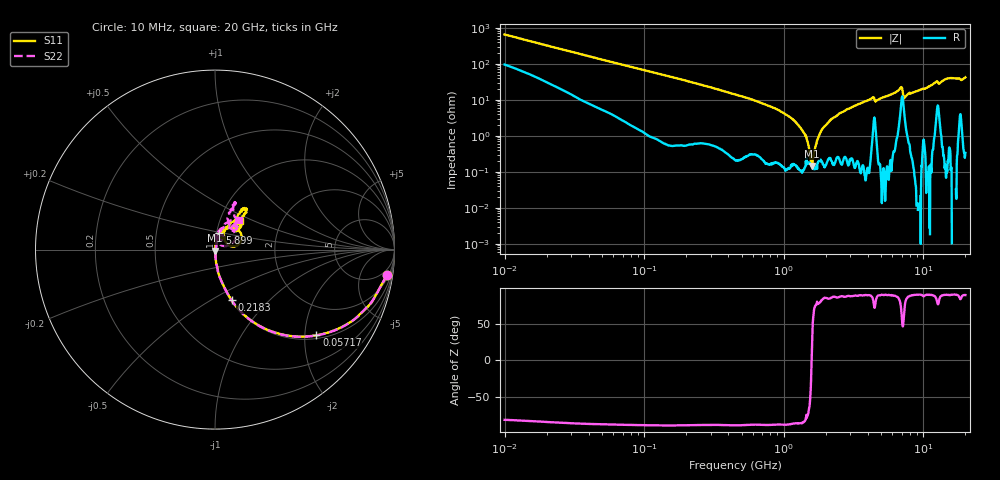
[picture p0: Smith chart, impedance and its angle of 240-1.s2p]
!Keysight Technologies,P5008B,MY61100088,A.16.20.02
!Date: Monday, May 27, 2024 17:33:43
!Correction: S11(C* 2-Port  )
!S21(C* 2-Port  )
!S12(C* 2-Port  )
!S22(C* 2-Port  )
!S2P File: Measurements: S11, S21, S12, S22:Log Frequency Sweep
# Hz S  dB  R 50
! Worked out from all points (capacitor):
!   1601 points, 10 MHz to 20 GHz, reference 50 ohm
!   read as one part in series: C = 24.8 pF near 10.39 MHz
!   lowest |Z| = 145 mohm at 1.59 GHz (marker M1)
!   series resonance near 1.582 GHz, so ESL is about 410 pH
!   S11 on the Smith chart (normalised r, x): 10 MHz: 3, -13; 57.17 MHz: 1.09, -2.29; 218.3 MHz: 1.01, -0.62; 5.899 GHz: 1.03, +0.19; 20 GHz: 1.24, +0.42
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1e7  -0.27 -8.5  -16.54 73.1  -16.55 73.1  -0.29 -8.5
3.555162e7  -1.33 -28.0  -6.53 58.9  -6.54 58.9  -1.34 -28.1
5.717073e7  -2.62 -40.2  -3.78 47.7  -3.79 47.7  -2.62 -40.3
1.263918e8  -6.62 -61.5  -1.14 27.8  -1.15 27.8  -6.61 -61.5
2.182631e8  -10.57 -71.9  -0.44 17.0  -0.45 17.0  -10.58 -71.9
4.472136e8  -16.93 -81.4  -0.11 7.9  -0.12 7.9  -16.94 -81.6
1.14013e9  -28.83 -85.4  -0.01 1.4  -0.02 1.4  -28.83 -85.0
1.438959e9  -35.07 -82.3  -0.00 0.1  -0.01 0.1  -34.59 -76.1
1.589917e9  -43.85 -82.3  0.00 -0.4  -0.01 -0.4  -41.55 -64.3
1.748386e9  -57.99 -29.6  0.00 -1.0  -0.01 -1.0  -45.46 -16.9
1.931805e9  -41.28 83.6  0.00 -1.5  -0.01 -1.5  -41.35 53.9
2.496738e9  -30.75 81.1  0.00 -3.1  -0.01 -3.1  -30.99 73.6
4.270791e9  -22.12 84.8  -0.06 -8.0  -0.07 -8.0  -21.48 70.6
4.652055e9  -24.30 85.4  -0.05 -7.4  -0.06 -7.4  -23.75 69.8
5.652411e9  -21.26 77.9  -0.02 -10.2  -0.03 -10.3  -21.31 79.3
5.899321e9  -20.51 75.3  -0.03 -10.9  -0.04 -10.9  -20.68 79.7
6.83533e9  -16.28 53.0  -0.40 -14.9  -0.41 -14.9  -16.98 63.8
7.445538e9  -22.79 38.4  -0.15 -10.7  -0.15 -10.7  -25.45 78.9
1.023592e10  -20.90 62.6  -0.04 -18.2  -0.05 -18.3  -21.10 71.4
1.482695e10  -11.16 55.7  -0.29 -27.9  -0.30 -27.9  -11.13 66.1
1.871311e10  -16.34 43.5  -0.25 -32.9  -0.26 -33.0  -16.93 49.0
2e10  -13.46 49.6  -0.16 -37.5  -0.17 -37.5  -13.37 51.0
